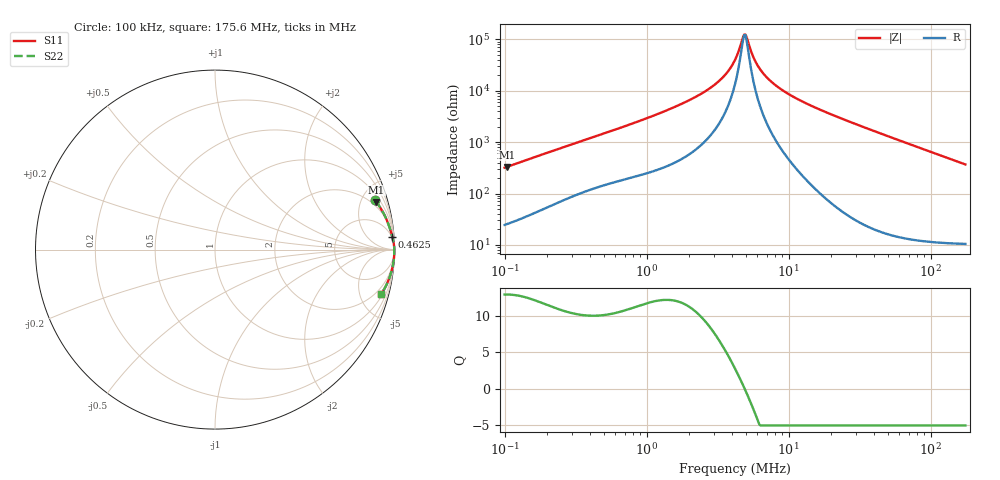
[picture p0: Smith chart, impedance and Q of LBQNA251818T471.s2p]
! LBQNA251818T471  S-PARAMETER MODEL  ( General Type )
! Model Generated by TAIYO YUDEN Corporation (http://www.ty-top.com)
! Version 1.0
! TAIYO YUDEN Control No. 191025NI43SB-FBB
! Copyright(c) 2019 TAIYO YUDEN CO.,LTD. All Rights Reserved.
! Product Description (link to TY-COMPAS)
! https://ds.yuden.co.jp/TYCOMPAS/or/detail?pn=LBQNA251818T471K&u=M
! Products Name : Inductors
! Characteristics :
!  Inductance : 470 uH , SRF(min) : 3.5 MHz , DC Resistance(max) : 13 Ohm
!  Rated Current : Saturation :35 mA , Temp Rise : 70 mA (20 degC)
!  Case Size : 2.5 x 1.8 / 0.098 x 0.071 [mm/inch] , Thickness : 1.8 / 0.071 [mm/inch]
!  (Conditions: Temperature = 25 degC , DC Bias Current/Voltage = 0A / 0V)
! External Node Assignments :
!  1  o---GGG---o  2
! GND o---------o GND
! Frequency Range : 0.1MHz  -  175.64884MHz  [ 402 STEP ]
# MHz S RI R 50
! Freq[MHz].  S11 Real  S11 Imag  S21 Real  S21 Imag  S12 Real  S12 Imag  S22 Real  S22 Imag
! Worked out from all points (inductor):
!   401 points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, 100 kHz to 175.6 MHz, reference 50 ohm
!   read as one part in series: L = 500 uH near 103.8 kHz
!   highest Q = 12.9 at 103.8 kHz (marker M1), where L = 503 uH
!   self-resonance near 4.866 MHz
!   S11 on the Smith chart (normalised r, x): 100 kHz: 1.49, +6.33; 462.5 kHz: 4, +27; 175.6 MHz: 1.21, -7.34
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0.1  0.8924 0.2736  0.1076 -0.2736  0.1076 -0.2736  0.8924 0.2736
0.103806  0.8985 0.2658  0.1015 -0.2658  0.1015 -0.2658  0.8985 0.2658
0.18871  0.9589 0.1603  0.0411 -0.1603  0.0411 -0.1603  0.9589 0.1603
0.349525  0.9821 0.0922  0.0179 -0.0922  0.0179 -0.0922  0.9821 0.0922
0.462543  0.9876 0.0716  0.0124 -0.0716  0.0124 -0.0716  0.9876 0.0716
1.221676  0.997 0.0276  0.00304 -0.0276  0.00304 -0.0276  0.997 0.0276
2.022878  0.9984 0.0149  0.00156 -0.0149  0.00156 -0.0149  0.9984 0.0149
2.884632  0.9989 0.0083  0.00109 -0.0083  0.00109 -0.0083  0.9989 0.0083
3.677404  0.9991 0.00438  0.000918 -0.00438  0.000918 -0.00438  0.9991 0.00438
3.962669  0.9991 0.00323  0.000879 -0.00323  0.000879 -0.00323  0.9991 0.00323
4.270063  0.9992 0.0021  0.000846 -0.0021  0.000846 -0.0021  0.9992 0.0021
4.776436  0.9992 0.000416  0.000805 -0.000416  0.000805 -0.000416  0.9992 0.000416
4.958236  0.9992 -0.000143  0.000794 0.000143  0.000794 0.000143  0.9992 -0.000143
5.146955  0.9992 -0.000702  0.000783 0.000702  0.000783 0.000702  0.9992 -0.000702
5.546217  0.9992 -0.00182  0.000766 0.00182  0.000766 0.00182  0.9992 -0.00182
5.86586  0.9992 -0.00267  0.000755 0.00267  0.000755 0.00267  0.9992 -0.00267
6.320889  0.9993 -0.00382  0.000743 0.00382  0.000743 0.00382  0.9993 -0.00382
7.070462  0.9993 -0.00559  0.000733 0.00559  0.000733 0.00559  0.9993 -0.00559
9.533088  0.9992 -0.0107  0.000751 0.0107  0.000751 0.0107  0.9992 -0.0107
14.64875  0.999 -0.02  0.000961 0.02  0.000961 0.02  0.999 -0.02
51.20104  0.9929 -0.078  0.0071 0.078  0.0071 0.078  0.9929 -0.078
175.6488  0.9249 -0.2498  0.0751 0.2498  0.0751 0.2498  0.9249 -0.2498
